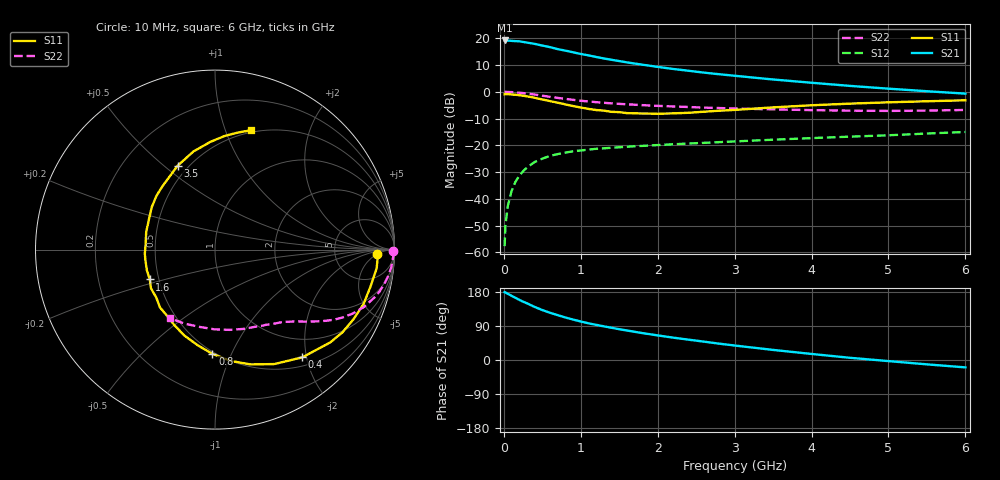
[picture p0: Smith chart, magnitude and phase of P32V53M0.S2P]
! SIEMENS Small Signal Semiconductors
! BFP181
! Si NPN RF Bipolar Junction Transistor in SOT143
! VCE = 2.5 V  IC = 3 mA
! Common Emitter S-Parameters:  March  1996
# GHz  S  MA  R  50
!  f  S11  S21  S12  S22
! GHz  MAG  ANG  MAG  ANG  MAG  ANG  MAG  ANG
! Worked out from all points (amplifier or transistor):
!   36 points, 10 MHz to 6 GHz, reference 50 ohm
!   highest |S21| = 19.2 dB at 10 MHz (marker M1)
!   |S21| within 3 dB of that: start of sweep to 668 MHz
!   unconditionally stable (mu >= 1): 2.065 GHz to end of sweep
!   at 250 MHz: K = 0.16, MSG = 24.2 dB, |S12| = -29.7 dB
!   at 1.4 GHz: K = 0.77, MSG = 16.4 dB, |S12| = -20.9 dB
!   at 6 GHz: K = 1.10, MAG = 5.3 dB, |S12| = -15.0 dB
!   lowest NFmin = 1.40 dB at 450 MHz
!   S11 on the Smith chart (normalised r, x): 10 MHz: 18, -4; 400 MHz: 0.65, -1.92; 800 MHz: 0.48, -0.85; 1.6 GHz: 0.45, -0.18; 3.5 GHz: 0.44, +0.56; 6 GHz: 0.48, +1.23
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0.01  0.9006 -1.5  9.122 179.0  0.0013 85.3  0.9945 -0.6
0.02  0.9076 -2.7  9.073 178.3  0.0031 85.0  0.997 -1.2
0.05  0.9066 -6.6  9.085 174.7  0.0072 88.1  0.9919 -3.0
0.1  0.8901 -13.6  8.97 169.5  0.0139 80.7  0.9867 -5.9
0.2  0.8634 -26.8  8.798 158.9  0.0268 74.8  0.962 -11.5
0.25  0.8466 -33.0  8.556 153.9  0.0327 71.2  0.9461 -14.3
0.4  0.7726 -51.0  7.872 140.1  0.0486 61.6  0.889 -21.1
0.5  0.7183 -62.6  7.325 131.8  0.0562 56.1  0.8462 -24.9
0.6  0.6701 -72.7  6.846 124.7  0.0634 52.1  0.8054 -28.0
0.7  0.6266 -81.9  6.283 118.3  0.0684 48.3  0.7695 -30.5
0.8  0.5814 -91.4  5.886 112.2  0.0731 45.0  0.7373 -32.5
0.9  0.5414 -100.3  5.488 106.7  0.0773 42.5  0.7083 -34.3
1.1  0.4792 -117.9  4.801 96.8  0.0832 38.3  0.659 -37.4
1.3  0.4449 -133.5  4.203 88.8  0.0879 35.2  0.623 -40.0
1.6  0.3996 -155.4  3.55 77.9  0.0938 32.2  0.585 -43.3
1.8  0.3925 -170.1  3.217 71.0  0.0975 30.9  0.5633 -45.6
2.2  0.3955 165.8  2.674 59.0  0.1045 28.8  0.5326 -50.5
2.8  0.4427 137.5  2.13 43.1  0.1146 26.4  0.4973 -58.8
3.5  0.5113 114.1  1.7 26.6  0.1272 23.8  0.4699 -70.1
4.5  0.601 92.4  1.29 5.8  0.1451 19.4  0.4442 -90.4
5.5  0.6657 78.7  1.025 -11.5  0.1659 15.5  0.4457 -112.2
6  0.695 73.1  0.924 -19.5  0.1776 12.6  0.4578 -123.4
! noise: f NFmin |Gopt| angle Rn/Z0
0.45  1.4  0.56  17  0.36
0.9  1.5  0.45  35  0.34
1.8  1.85  0.25  82  0.36
